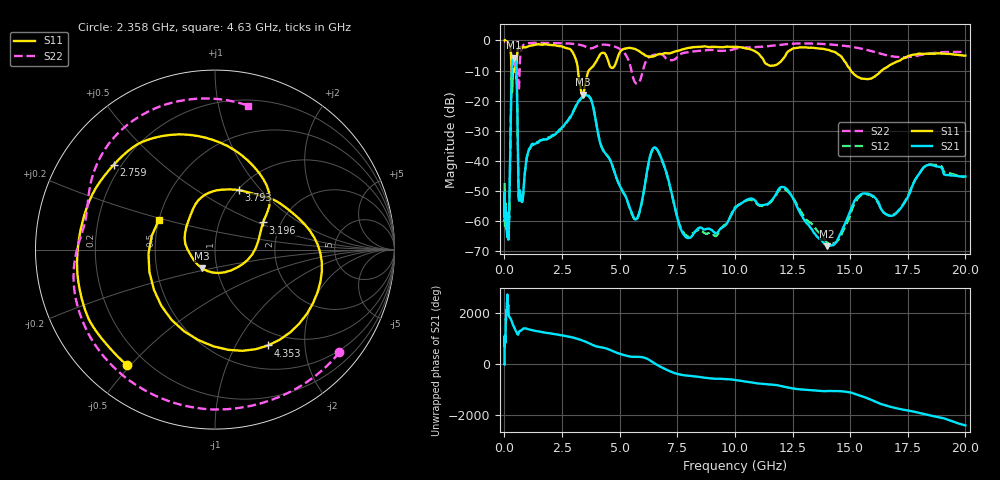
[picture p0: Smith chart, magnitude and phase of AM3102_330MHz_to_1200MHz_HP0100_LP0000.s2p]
! Date/Time: Tue, Sep 11, 2018 5:12 PM
! Network Analyzer: Agilent Technologies E8362B Rev: A.07.50.63
! Sweep from 0.010 to 20.000 GHz, 1601 Points, Sweep Type: LOG
! Power Supply: 4.949 V, 0.000 A
# Hz S DB R 50
!freq MagS11 AngS11 MagS21 AngS21 MagS12 AngS12 MagS22 AngS22
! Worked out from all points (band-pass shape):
!   1601 points, 10 MHz to 20 GHz, reference 50 ohm
!   highest |S21| = -5.73 dB at 412.5 MHz (marker M1); lowest = -68.3 dB at 14.01 GHz (marker M2)
!   |S21| within 3 dB of the highest: 329.3 MHz to 514.4 MHz (185.1 MHz wide, 43.9 % of centre)
!   lowest |S11| = -18.0 dB at 3.4 GHz (marker M3), VSWR 1.29, Z = 42.5 - j9.02 ohm
!   |S11| at or under -10 dB: 308 MHz to 364.5 MHz (56.5 MHz wide, 16.8 % of centre); 3.193 GHz to 3.663 GHz (469.7 MHz wide, 13.7 % of centre); 15.03 GHz to 16.37 GHz (1.344 GHz wide, 8.56 % of centre)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
!   |S22| runs from -16.6 to -0.2 dB; largest |S21 - S12| = 0.006
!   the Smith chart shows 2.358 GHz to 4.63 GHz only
!   S11 on the Smith chart (normalised r, x): 2.358 GHz: 0.13, -0.49; 2.759 GHz: 0.17, +0.35; 3.196 GHz: 1.62, +0.54; 3.793 GHz: 1.01, +0.77; 4.353 GHz: 0.80, -1.37; 4.63 GHz: 0.50, +0.19
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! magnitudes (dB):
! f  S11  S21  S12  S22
! 10 MHz  0.0  -54.2  -47.4  -0.2
! 35.55 MHz  0.0  -58.3  -57.3  -0.3
! 126.4 MHz  -0.4  -64.6  -64.1  -0.7
! 199.4 MHz  -1.1  -59.9  -61.3  -1.3
! 412.5 MHz  -10.4  -5.7  -5.8  -7.4
! 447.2 MHz  -9.4  -6.0  -6.1  -7.3
! 530.6 MHz  -7.3  -11.6  -11.6  -12.5
! 635.6 MHz  -2.3  -53.2  -53.6  -15.9
! 1.59 GHz  -1.4  -33.1  -33.1  -0.8
! 2.358 GHz  -1.8  -29.9  -30.3  -0.9
! 2.759 GHz  -2.7  -26.6  -26.6  -1.0
! 3.196 GHz  -10.3  -20.4  -20.6  -1.3
! 3.4 GHz  -18.0  -18.5  -18.7  -1.7
! 3.793 GHz  -8.9  -20.4  -20.3  -2.6
! 4.353 GHz  -4.3  -37.2  -37.1  -1.4
! 4.63 GHz  -9.0  -40.4  -40.5  -1.7
! 5.652 GHz  -2.8  -59.3  -59.5  -13.7
! 6.58 GHz  -4.9  -35.8  -35.9  -4.6
! 7.882 GHz  -2.6  -65.4  -64.7  -4.0
! 12.09 GHz  -6.1  -48.7  -49.2  -1.4
! 14.01 GHz  -3.1  -68.3  -67.2  -1.3
! 20 GHz  -5.0  -45.2  -45.4  -3.8
